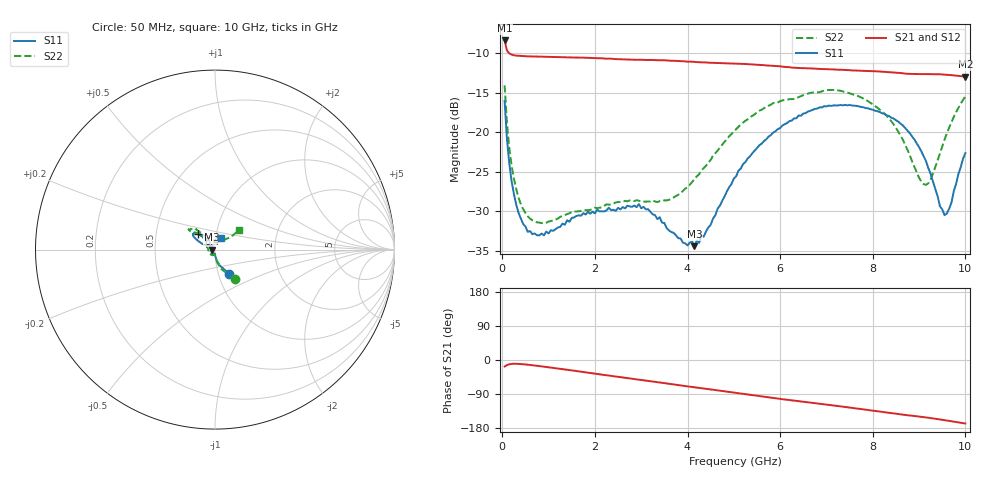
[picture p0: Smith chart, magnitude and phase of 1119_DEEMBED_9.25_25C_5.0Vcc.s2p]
!Hittite Microwave Corp.
!Digital Attenuator/PhaseShifter Rev 1.4.0
!Filename: C:\DATA\DATA\1119_DEEMBED_9.25_25C_5.0Vcc.s2p
!VNA ID: Agilent Technologies,N5224A,MY51441122,A.10.45.03
!Device type:
!2 Port Calibration.
!Temp(C): 25
!Lot Number:
!Serial Number:
!Operator:
!Misc:
!Attenuator:  9.250
# GHZ S DB R 50.0
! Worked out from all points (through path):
!   200 points, 50 MHz to 10 GHz, reference 50 ohm
!   highest |S21| = -8.36 dB at 50 MHz (marker M1); lowest = -12.9 dB at 10 GHz (marker M2)
!   group delay of S21, straight-line fit = 45 ps
!   lowest |S11| = -34.4 dB at 4.15 GHz (marker M3), VSWR 1.04, Z = 48.1 - j0.116 ohm
!   |S11| at or under -10 dB: start of sweep to end of sweep
!   |S22| runs from -31.5 to -14.0 dB; largest |S21 - S12| = 0.00077
!   S11 on the Smith chart (normalised r, x): 50 MHz: 1.13, -0.32; 6.4 GHz: 0.82, +0.15; 10 GHz: 1.06, +0.14
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0.05  -16.00 -59.4  -8.36 -17.2  -8.35 -17.3  -14.03 -56.3
0.1  -20.79 -73.6  -9.62 -13.6  -9.61 -13.6  -18.76 -71.6
0.15  -23.84 -79.7  -9.99 -11.3  -9.99 -11.3  -21.91 -78.2
0.25  -27.75 -85.4  -10.23 -9.9  -10.23 -10.0  -25.83 -84.4
0.4  -30.88 -90.7  -10.33 -10.7  -10.33 -10.7  -29.09 -88.5
0.55  -32.58 -94.2  -10.37 -12.4  -10.36 -12.4  -30.61 -91.5
0.9  -33.03 -100.9  -10.42 -17.6  -10.42 -17.6  -31.47 -97.0
1.75  -30.21 -114.4  -10.54 -31.7  -10.55 -31.7  -29.84 -109.9
2.95  -29.08 -118.0  -10.80 -51.6  -10.81 -51.6  -28.65 -147.5
3.4  -30.73 -129.8  -10.86 -59.3  -10.87 -59.3  -28.69 -168.0
4.15  -34.39 -176.4  -11.08 -72.1  -11.08 -72.2  -25.93 152.3
5.05  -25.55 136.1  -11.30 -86.7  -11.32 -86.7  -19.59 130.5
5.55  -21.62 134.1  -11.46 -95.2  -11.47 -95.2  -17.24 131.3
6.4  -17.85 136.3  -11.85 -108.6  -11.86 -108.6  -15.53 137.5
6.7  -17.14 138.7  -11.91 -113.1  -11.92 -113.1  -14.95 139.8
7.65  -16.64 146.6  -12.17 -127.9  -12.17 -127.9  -15.31 143.5
8.35  -17.92 150.3  -12.36 -139.3  -12.36 -139.3  -18.23 133.9
8.75  -19.74 153.1  -12.58 -145.7  -12.57 -145.7  -22.21 120.2
9.15  -23.64 155.4  -12.62 -151.6  -12.63 -151.6  -26.63 82.7
9.55  -30.46 114.5  -12.68 -158.8  -12.69 -158.8  -20.89 42.5
9.7  -28.87 82.1  -12.75 -161.7  -12.76 -161.7  -18.70 38.9
10  -22.60 62.7  -12.94 -167.6  -12.95 -167.5  -15.44 39.1
